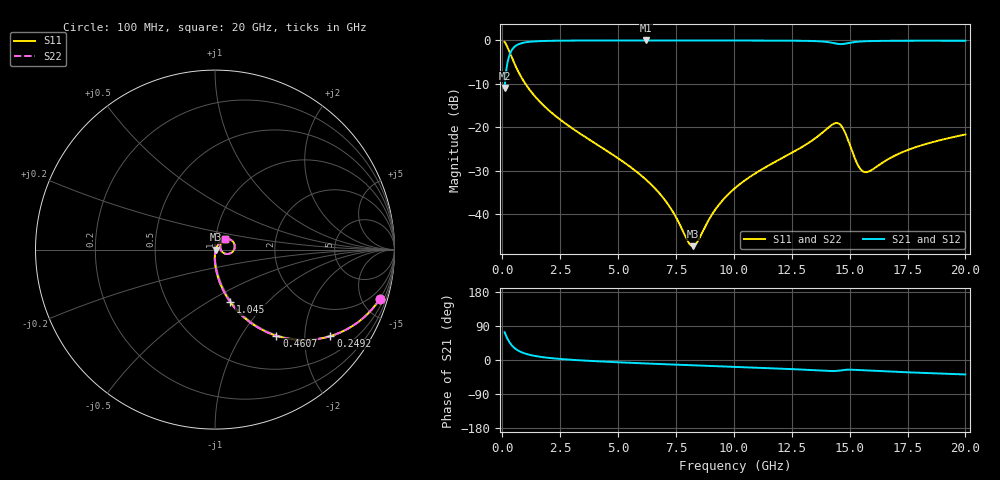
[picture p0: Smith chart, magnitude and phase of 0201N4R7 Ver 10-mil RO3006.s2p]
# GHz S MA R 50
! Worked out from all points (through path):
!   1601 points, 100 MHz to 20 GHz, reference 50 ohm
!   highest |S21| = -0.04 dB at 6.207 GHz (marker M1); lowest = -10.9 dB at 100 MHz (marker M2)
!   group delay of S21, straight-line fit = 7.6 ps
!   lowest |S11| = -47.3 dB at 8.222 GHz (marker M3), VSWR 1.01, Z = 50.4 - j0.123 ohm
!   |S11| at or under -10 dB: 998.3 MHz to end of sweep
!   |S22| runs from -47.3 to -0.4 dB; largest |S21 - S12| = 0
!   S11 on the Smith chart (normalised r, x): 100 MHz: 0.98, -6.69; 249.2 MHz: 0.98, -2.68; 460.7 MHz: 0.98, -1.45; 1.045 GHz: 0.98, -0.63; 20 GHz: 1.11, +0.13
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0.1  0.9587 -16.7  0.2838 73.3  0.2838 73.3  0.9587 -16.7
0.24925  0.8039 -36.8  0.5937 53.1  0.5937 53.1  0.8039 -36.8
0.4606875  0.5896 -54.5  0.8064 35.3  0.8064 35.3  0.5896 -54.5
0.697  0.4333 -65.3  0.8999 24.5  0.8999 24.5  0.4333 -65.3
1.04525  0.303 -73.9  0.9514 15.9  0.9514 15.9  0.303 -73.9
1.978063  0.1594 -83.5  0.9851 5.8  0.9851 5.8  0.1594 -83.5
3.420812  0.08258 -89.2  0.9938 -1.1  0.9938 -1.1  0.08258 -89.2
6.206812  0.02503 -90.8  0.9959 -9.2  0.9959 -9.2  0.02503 -90.8
6.741625  0.01801 -88.2  0.9959 -10.5  0.9959 -10.5  0.01801 -88.2
8.221687  0.004305 -16.4  0.9955 -14.0  0.9955 -14.0  0.004305 -16.4
8.420687  0.004804 10.1  0.9954 -14.4  0.9954 -14.4  0.004804 10.1
9.254  0.01187 50.4  0.995 -16.3  0.995 -16.3  0.01187 50.4
10.05  0.02001 57.2  0.9945 -18.2  0.9945 -18.2  0.02001 57.2
13.37081  0.07024 50.9  0.982 -26.5  0.982 -26.5  0.07024 50.9
14.47775  0.1118 10.9  0.9108 -28.5  0.9108 -28.5  0.1118 10.9
14.73894  0.09448 -10.1  0.9086 -26.4  0.9086 -26.4  0.09448 -10.1
15.29862  0.0397 -15.4  0.9606 -26.2  0.9606 -26.2  0.0397 -15.4
15.55981  0.03135 2.3  0.9722 -27.1  0.9722 -27.1  0.03135 2.3
15.85831  0.03128 22.0  0.9793 -28.1  0.9793 -28.1  0.03128 22.0
16.69162  0.04345 43.2  0.9865 -30.5  0.9865 -30.5  0.04345 43.2
18.02244  0.06113 47.7  0.9886 -33.7  0.9886 -33.7  0.06113 47.7
20  0.08274 46.2  0.988 -38.2  0.988 -38.2  0.08274 46.2
